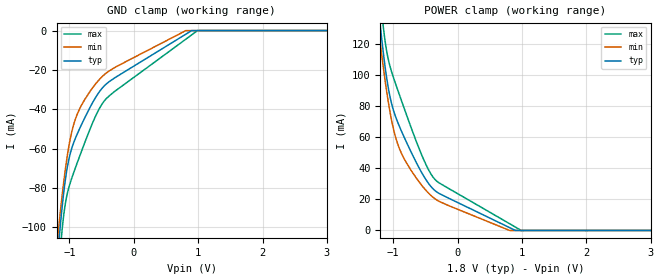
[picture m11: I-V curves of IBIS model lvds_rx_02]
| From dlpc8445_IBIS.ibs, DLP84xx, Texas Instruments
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|   MODEL lvds_rx_02
[Model] lvds_rx_02
Model_type Input
C_comp 1.395p 1.496p 1.31p
Vinl = 1.1
Vinh = 1.3
[Model Spec]
[Temperature Range]  40 150 -40
[Voltage Range] 1.8 1.62 1.98
[GND Clamp]
-1.753V   -392.3mA   -335.2mA   -469.7mA
-1.174V   -111.2mA   -102.7mA   -125.5mA
-1.148V   -101.6mA   -94.46mA   -114.3mA
-1.112V   -89.43mA   -83.63mA   -100.9mA
-1.035V   -69.98mA   -64.16mA   -83.19mA
-907.2mV  -54.76mA   -45mA      -69.76mA
-758.6mV  -44.12mA   -34.86mA   -56.64mA
-548.4mV  -31.73mA   -25.34mA   -40.45mA
-297.2mV  -24.03mA   -18.79mA   -30.91mA
810mV     -1.81mA    0A         -4.336mA
990mV     0A         0A         0A
3.548V    0A         0A         0A
[Power Clamp]
-1.753V   400mA      343.8mA    476.2mA
-1.225V   142.5mA    129.7mA    162.5mA
-1.189V   128.1mA    117.3mA    145.9mA
-1.148V   113.1mA    103.9mA    129.6mA
-1.097V   97.4mA     88.7mA     114.8mA
-1.041V   84.65mA    74.58mA    104.7mA
-897mV    66.58mA    52.25mA    86.83mA
-517.7mV  34.57mA    27.17mA    44.98mA
-307.5mV  24.41mA    19.28mA    31.31mA
810mV     1.811mA    0A         4.336mA
990mV     0A         0A         0A
3.553V    0A         0A         0A
